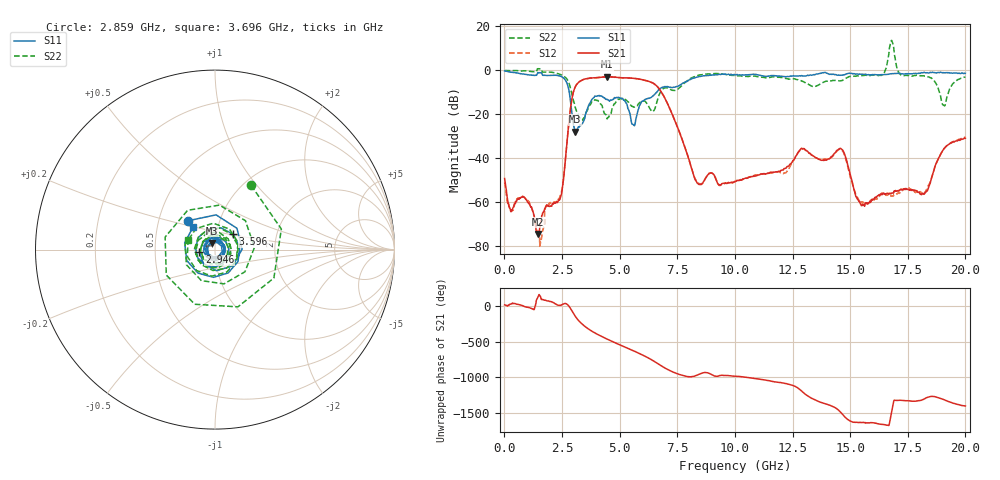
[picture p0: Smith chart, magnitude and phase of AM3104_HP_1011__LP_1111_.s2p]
!Created with skrf (http://scikit-rf.org).
# Hz S RI R 50.0
!freq ReS11 ImS11 ReS21 ImS21 ReS12 ImS12 ReS22 ImS22
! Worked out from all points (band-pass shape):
!   1601 points, 10 MHz to 20 GHz, reference 50 ohm
!   highest |S21| = -2.90 dB at 4.458 GHz (marker M1); lowest = -74.3 dB at 1.447 GHz (marker M2)
!   |S21| within 3 dB of the highest: 3.175 GHz to 6.472 GHz (3.297 GHz wide, 68.4 % of centre)
!   lowest |S11| = -27.8 dB at 3.071 GHz (marker M3), VSWR 1.09, Z = 48.1 + j3.52 ohm
!   |S11| at or under -10 dB: 2.816 GHz to 6.601 GHz (3.785 GHz wide, 80.4 % of centre)
!   |S22| runs from -22.7 to 13.6 dB; largest |S21 - S12| = 0.083
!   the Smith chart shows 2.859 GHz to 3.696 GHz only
!   S11 on the Smith chart (normalised r, x): 2.859 GHz: 0.71, +0.24; 2.946 GHz: 0.84, -0.02; 3.596 GHz: 1.20, +0.21; 3.696 GHz: 0.76, +0.20
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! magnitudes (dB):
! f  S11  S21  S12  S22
! 10 MHz  -0.2  -49.1  -50.8  0.0
! 259.9 MHz  -0.8  -63.0  -63.7  -0.1
! 1.447 GHz  -1.0  -74.3  -74.1  0.8
! 2.446 GHz  -2.7  -57.3  -56.3  -1.9
! 2.859 GHz  -13.2  -18.0  -18.1  -7.7
! 2.946 GHz  -21.1  -12.0  -12.1  -11.5
! 3.071 GHz  -27.8  -7.6  -7.6  -16.6
! 3.346 GHz  -24.4  -4.5  -4.6  -22.6
! 3.596 GHz  -17.6  -3.6  -3.7  -18.2
! 3.696 GHz  -15.1  -3.4  -3.5  -15.9
! 4.458 GHz  -13.1  -2.9  -2.9  -22.1
! 5.607 GHz  -24.8  -3.6  -3.6  -16.6
! 6.682 GHz  -8.9  -7.8  -7.9  -12.0
! 8.368 GHz  -3.0  -51.2  -50.7  -2.3
! 10.01 GHz  -2.0  -50.6  -50.4  -2.4
! 13.34 GHz  -2.2  -38.5  -38.6  -7.2
! 14.64 GHz  -2.2  -35.9  -36.2  -4.6
! 15.54 GHz  -1.7  -61.4  -60.3  -2.3
! 16.68 GHz  -1.7  -56.0  -56.8  7.3
! 18.26 GHz  -1.1  -55.5  -55.2  -2.6
! 19.05 GHz  -1.0  -35.9  -35.9  -15.8
! 20 GHz  -1.3  -30.8  -30.4  -3.0
